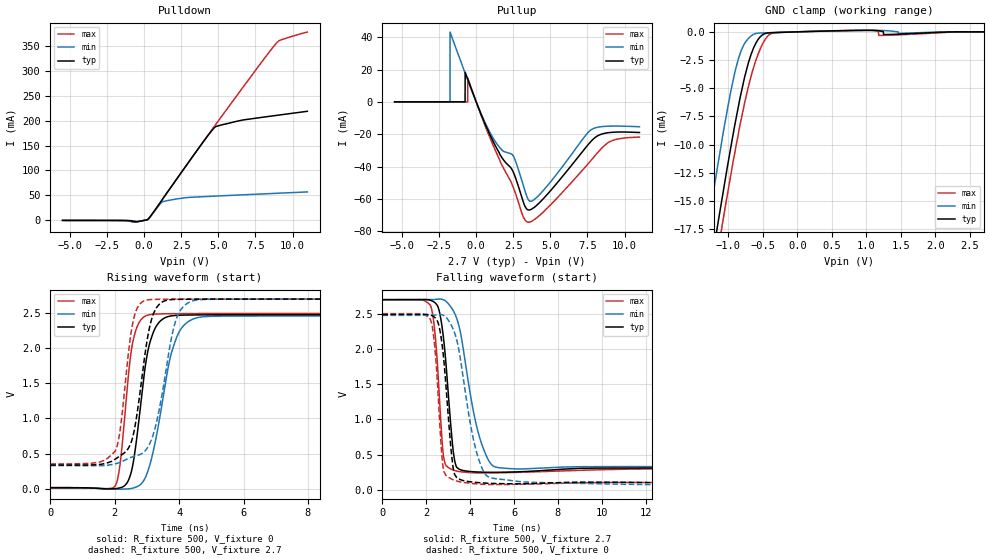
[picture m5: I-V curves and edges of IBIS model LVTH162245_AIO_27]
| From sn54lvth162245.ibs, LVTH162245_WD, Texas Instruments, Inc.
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[Model]   LVTH162245_AIO_27
Model_type  I/O
Vinl = 0.8
Vinh = 2.0
Enable   Active-Low
Vref =   0
Rref =   500
Cref =   50p
Vmeas =   1.5
| variable   typ   min   max
C_comp   10.0pF   NA   NA
| C_pullup   1.94pF   1.15pF   3.08pF
| C_pulldown   4.40pF   3.60pF   4.89pF
| C_tri-state   5.34pF   4.19pF   6.43pF
[Temperature Range]   40   -40   100
| Ambient temperature   25   -40   85
[Voltage range]   2.7   2.7   2.7
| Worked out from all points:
|   slope of the pulldown table from 0 to 0.405 V, typ, clamps not added: 55 ohm
|   slope of the pullup table from 0 to 0.405 V, typ, clamps not added: 43.1 ohm
|   GND clamp passes 1 mA (typ) near -0.60 V on its own axis
|   rising waveform, R_fixture 500, V_fixture 0: 20-80 % time 420ps typ, 606ps min, 320ps max; typ from 0.012 V to 2.48 V
|   falling waveform, R_fixture 500, V_fixture 2.7: 20-80 % time 392ps typ, 815ps min, 300ps max; typ from 2.7 V to 0.328 V
|   rising waveform, R_fixture 500, V_fixture 2.7: 20-80 % time 453ps typ, 581ps min, 348ps max; typ from 0.337 V to 2.7 V
|   falling waveform, R_fixture 500, V_fixture 0: 20-80 % time 402ps typ, 833ps min, 311ps max; typ from 2.49 V to 0.015 V
[GND Clamp]
| LVTH162245_AIO_27
|   Voltage   I(typ)   I(min)   I(max)
-5.5V     -196.4mA   -192.8mA   -198.3mA
-1.3V     -22.73mA   -17.52mA   -25.18mA
-1.145V   -16.83mA   -11.6mA    -19.29mA
-1.07V    -14.07mA   -8.833mA   -16.52mA
-970mV    -10.5mA    -5.486mA   -12.94mA
-850mV    -6.523mA   -2.324mA   -8.923mA
-775mV    -4.351mA   -1.156mA   -6.651mA
-670mV    -2.009mA   -368.1uA   -3.957mA
-510mV    -293.9uA   -97.94uA   -1.166mA
-415mV    -94.27uA   -77.91uA   -296.1uA
-300mV    -59.35uA   -55.07uA   -73.82uA
2.7V      25.88pA    18.5pA     1.8nA
[Pulldown]
| LVTH162245_AIO_27
|   Voltage   I(typ)   I(min)   I(max)
-5.5V     -55.1uA    -362.1uA   -90.08uA
-1.46V    -381.6uA   -457.7uA   -209.7uA
-685mV    -2.27mA    -3.713mA   -1.345mA
265mV     2.265mA    2.576mA    1.916mA
1.265V    43.61mA    37.39mA    43.26mA
2.85V     110.2mA    45.56mA    110.5mA
4.285V    169.3mA    47.84mA    170mA
4.795V    187.2mA    48.59mA    190.9mA
6.615V    200.9mA    51.1mA     264.8mA
8.98V     210.6mA    54.27mA    357.3mA
9.27V     211.8mA    54.66mA    362.2mA
11V       218.6mA    56.94mA    377.4mA
[Pullup]
| LVTH162245_AIO_27
|   Voltage   I(typ)   I(min)   I(max)
-5.5V     57.02uA    34.21uA    93.15uA
-1.765V   50.15uA    311uA      80.15uA
-1.76V    50.14uA    43.18mA    80.13uA
-750mV    35.59uA    17.91mA    73.97uA
-745mV    18.36mA    17.79mA    73.66uA
-570mV    14mA       13.53mA    41.33uA
-565mV    13.87mA    13.41mA    14.64mA
1.16V     -24.77mA   -22.64mA   -27.22mA
2.515V    -43.73mA   -33.64mA   -53.15mA
3.465V    -66.59mA   -59.51mA   -74.27mA
7.765V    -24.11mA   -17.06mA   -35.84mA
11V       -18.88mA   -15.33mA   -21.7mA
[Ramp]
| LVTH162245_AIO_27
| variable   typ   min   max
dV/dt_r   1.49/4.28E-10   1.48/6.17E-10   1.50/3.25E-10
dV/dt_f   1.47/4.08E-10   1.45/8.40E-10   1.48/3.12E-10
R_load = 500
[Rising Waveform]
| LVTH162245_AIO_27
R_fixture =   500
C_fixture =   0
L_fixture =   0
V_fixture =   0
V_fixture_min = 0
V_fixture_max = 0
|   Time   V(typ)   V(min)   V(max)
0s        12.4mV     7.922mV    15.85mV
2.01ns    -1.374mV   -5.754mV   33.4mV
2.17ns    12.44mV    -7.421mV   361.2mV
2.39ns    87.28mV    -3.636mV   1.433V
2.67ns    668.3mV    23.46mV    2.275V
2.96ns    1.776V     166.9mV    2.459V
3.175ns   2.197V     489.3mV    2.483V
3.9ns     2.467V     2.127V     2.492V
4.755ns   2.475V     2.449V     2.494V
50ns      2.478V     2.461V     2.495V
[Falling Waveform]
| LVTH162245_AIO_27
R_fixture =   500
C_fixture =   0
L_fixture =   0
V_fixture =   2.7
V_fixture_min = 2.7
V_fixture_max = 2.7
|   Time   V(typ)   V(min)   V(max)
0s        2.7V       2.7V       2.7V
2.17ns    2.693V     2.702V     2.628V
2.345ns   2.669V     2.703V     2.376V
2.525ns   2.605V     2.707V     1.709V
2.815ns   2.072V     2.694V     429.1mV
3.23ns    546.2mV    2.544V     281.8mV
3.505ns   292.3mV    2.307V     260.3mV
4.4ns     253mV      776.8mV    240.4mV
5.31ns    250mV      314.4mV    242.1mV
50ns      327.9mV    328.5mV    343.2mV
[Rising Waveform]
| LVTH162245_AIO_27
R_fixture =   500
C_fixture =   0
L_fixture =   0
V_fixture =   2.7
V_fixture_min = 2.7
V_fixture_max = 2.7
|   Time   V(typ)   V(min)   V(max)
0s        336.6mV    328.7mV    352.8mV
2.01ns    418.2mV    352.7mV    532.2mV
2.17ns    467.6mV    374.2mV    841mV
2.435ns   584.2mV    433.3mV    1.968V
2.58ns    771.7mV    456.1mV    2.401V
3.07ns    2.272V     626.3mV    2.691V
3.37ns    2.619V     1.098V     2.696V
3.91ns    2.696V     2.413V     2.699V
4.62ns    2.699V     2.691V     2.7V
50ns      2.7V       2.7V       2.7V
[Falling Waveform]
| LVTH162245_AIO_27
R_fixture =   500
C_fixture =   0
L_fixture =   0
V_fixture =   0
V_fixture_min = 0
V_fixture_max = 0
|   Time   V(typ)   V(min)   V(max)
0s        2.489V     2.478V     2.502V
2.17ns    2.482V     2.479V     2.428V
2.51ns    2.396V     2.486V     1.515V
2.8ns     1.841V     2.475V     265.8mV
3.23ns    302.3mV    2.278V     142.9mV
3.675ns   132.8mV    1.61V      107.4mV
4.14ns    110mV      730.8mV    88.88mV
4.6ns     98.12mV    268.5mV    79.15mV
6.135ns   85.88mV    121.4mV    78.39mV
50ns      14.76mV    10.01mV    19.28mV
